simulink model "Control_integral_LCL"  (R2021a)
settings: Solver=ode45  StartTime=0.0  StopTime=0.08  MaxStep=1e-4  RelTol=1e-3  EnableMultiTasking=on
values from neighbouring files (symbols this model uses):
  A = [0 0 -1/L;0 0 1/L;1/Cf -1/Cf 0]    [LCL_int2.m]
  B = [1/L;0;0]    [LCL_int2.m]
undefined symbols (not defined in the file or in its folder): Kf

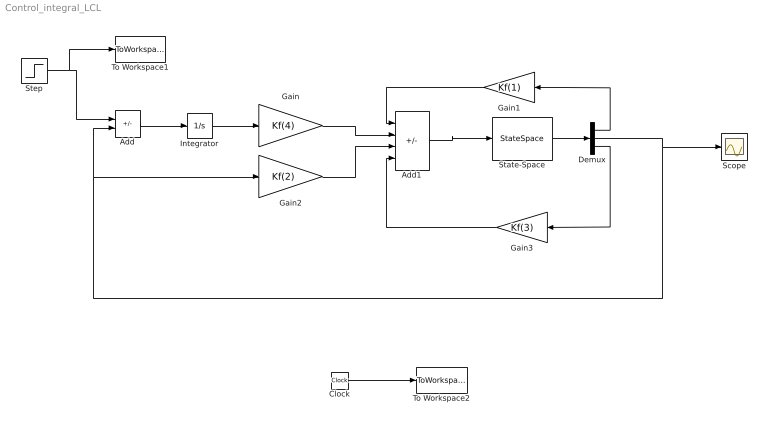
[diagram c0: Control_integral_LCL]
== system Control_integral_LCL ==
  Add : Sum  Inputs=-+
  Add1 : Sum  Inputs=----
  Clock : Clock
  Demux : Demux  Outputs=3
  Gain : Gain  Gain=Kf(4)
  Gain1 : Gain  Gain=Kf(1)
  Gain2 : Gain  Gain=Kf(2)
  Gain3 : Gain  Gain=Kf(3)
  Integrator : Integrator
  Scope : Scope
  State-Space : StateSpace  A=A  B=B  C=[1 0 0 ;0 1 0 ;0 0 1 ]  D=[0;0;0]  InitialCondition=0
  Step : Step  Time=0.01  After=10  SampleTime=0
  To Workspace1 : ToWorkspace  VariableName=in  SampleTime=-1
  To Workspace2 : ToWorkspace  VariableName=time  SampleTime=-1
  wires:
  Step/1 -> To Workspace1/1, Add/1
  Add/1 -> Integrator/1
  Integrator/1 -> Gain/1
  Add1/1 -> State-Space/1
  State-Space/1 -> Demux/1
  Demux/1 -> Gain1/1
  Demux/2 -> Gain2/1, Add/2, Scope/1
  Clock/1 -> To Workspace2/1
  Gain/1 -> Add1/2
  Gain1/1 -> Add1/1
  Gain2/1 -> Add1/3
  Gain3/1 -> Add1/4
  Demux/3 -> Gain3/1
